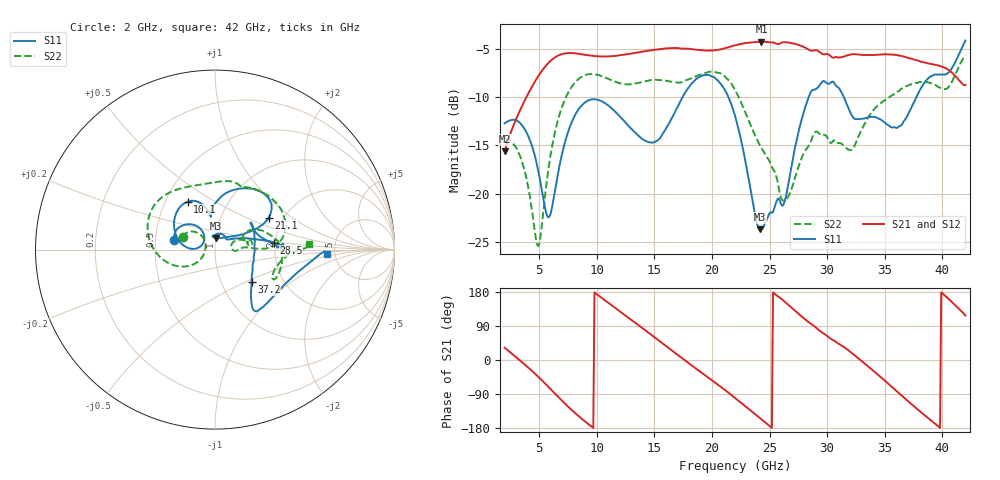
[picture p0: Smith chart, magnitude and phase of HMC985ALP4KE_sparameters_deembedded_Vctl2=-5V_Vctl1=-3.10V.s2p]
!s2p File: Measurements: S11, S21, S12, S22
# GHz S dB R 50.0
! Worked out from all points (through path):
!   401 points, 2 GHz to 42 GHz, reference 50 ohm
!   highest |S21| = -4.20 dB at 24.3 GHz (marker M1); lowest = -15.6 dB at 2 GHz (marker M2)
!   lowest |S11| = -23.7 dB at 24.2 GHz (marker M3), VSWR 1.14, Z = 50.3 + j6.53 ohm
!   |S11| at or under -10 dB: start of sweep to 17.43 GHz; 21.44 GHz to 28.39 GHz (6.948 GHz wide, 27.9 % of centre); 31.46 GHz to 37.74 GHz (6.275 GHz wide, 18.1 % of centre)
!   |S22| runs from -25.5 to -5.6 dB; largest |S21 - S12| = 0.00085
!   S11 on the Smith chart (normalised r, x): 2 GHz: 0.63, +0.07; 10.1 GHz: 0.65, +0.38; 21.1 GHz: 1.68, +0.68; 28.5 GHz: 1.96, +0.17; 37.2 GHz: 1.39, -0.54; 42 GHz: 4.32, -0.38
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2  -12.69 167.2  -15.59 32.5  -15.60 32.5  -14.25 158.8
3.5  -12.88 144.1  -10.92 -5.4  -10.92 -5.4  -16.64 138.2
4.9  -17.50 124.7  -7.82 -43.6  -7.83 -43.6  -25.48 172.8
5.9  -22.39 157.2  -6.29 -73.9  -6.29 -73.9  -16.65 -145.7
7.1  -15.30 173.3  -5.45 -111.0  -5.45 -111.0  -10.61 -169.1
8.7  -10.82 140.9  -5.50 -155.2  -5.51 -155.2  -7.84 156.9
10.1  -10.24 119.7  -5.72 171.3  -5.72 171.3  -7.65 134.5
13  -13.27 99.8  -5.43 106.1  -5.43 106.1  -8.61 96.0
15.4  -14.35 97.6  -4.99 51.2  -4.99 51.2  -8.18 73.1
18  -8.91 70.1  -4.93 -8.8  -4.94 -8.8  -8.10 61.3
21.1  -9.18 30.6  -4.88 -78.4  -4.88 -78.4  -7.79 16.1
22  -11.89 26.9  -4.57 -100.0  -4.58 -100.0  -9.21 5.2
24.2  -23.74 83.3  -4.21 -154.2  -4.21 -154.1  -15.06 4.0
24.3  -23.73 88.9  -4.20 -156.7  -4.20 -156.6  -15.27 4.3
26.3  -20.86 38.5  -4.25 154.0  -4.25 154.0  -20.74 10.5
28.5  -9.64 6.6  -5.10 97.7  -5.10 97.7  -14.85 16.8
28.7  -9.24 3.3  -5.14 93.7  -5.14 93.7  -14.19 16.4
32.4  -12.23 24.4  -5.50 11.8  -5.50 11.8  -14.98 27.1
35.4  -12.95 10.6  -5.51 -65.0  -5.51 -65.0  -9.98 14.9
37.2  -11.33 -41.3  -5.92 -113.3  -5.92 -113.3  -8.66 0.3
39.7  -7.60 -50.8  -6.68 -176.4  -6.69 -176.3  -8.94 -26.6
42  -4.07 -2.5  -8.70 117.2  -8.71 117.2  -5.60 3.4
